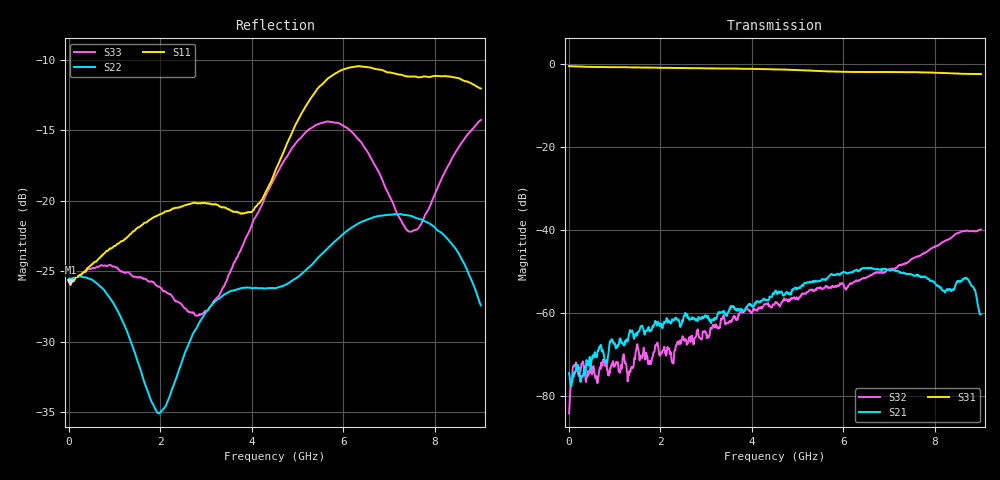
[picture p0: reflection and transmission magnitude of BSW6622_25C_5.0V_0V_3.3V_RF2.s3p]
!Agilent Technologies,N5230C,MY49001333,A.09.33.09
!Agilent N5230C: A.09.33.09
!Date: Monday, September 23, 2024 11:09:14
!Correction: S11(Full 3 Port(1,2,3))
!S12(Full 3 Port(1,2,3))
!S13(Full 3 Port(1,2,3))
!S21(Full 3 Port(1,2,3))
!S22(Full 3 Port(1,2,3))
!S23(Full 3 Port(1,2,3))
!S31(Full 3 Port(1,2,3))
!S32(Full 3 Port(1,2,3))
!S33(Full 3 Port(1,2,3))
!S3P File: Measurements: <S11,S12,S13>,
!<S21,S22,S23>,
!<S31,S32,S33>:
# Hz S  MA  R 50
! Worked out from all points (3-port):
!   901 points, 10 MHz to 9.01 GHz, reference 50 ohm
!   strongest paths, dB at 10 MHz, 2.26 GHz, 4.51 GHz, 6.76 GHz, 9.01 GHz:
!     S31: -0.6, -1.0, -1.3, -2.0, -2.5
!     S21: -74.4, -61.5, -54.7, -49.5, -60.2
!     S32: -84.1, -71.7, -57.6, -50.2, -39.9
!   lowest |S11| = -25.8 dB at 40 MHz (marker M1), VSWR 1.11, Z = 55.4 - j0.441 ohm
!   |S11| at or under -10 dB: start of sweep to end of sweep
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1e7  0.05148 -0.6  0.000127 11.6  0.9374 -2.5
     0.0001906 -47.2  0.05292 -1.2  9.816e-05 -60.5
     0.9373 -2.5  6.264e-05 -70.1  0.05153 -4.2
4e7  0.05144 -4.4  0.0001566 70.6  0.936 -4.7
     0.000147 -49.8  0.05296 -2.2  0.0001338 -132.6
     0.9357 -4.6  0.0001239 -5.2  0.05276 -3.4
1.6e9  0.08205 169.2  0.0006582 -76.7  0.9007 -167.9
       0.0007064 -62.9  0.02431 -139.4  0.0002741 -173.5
       0.9019 -168.0  0.0002947 -13.1  0.05339 175.8
2.63e9  0.0973 66.8  0.0008158 -164.1  0.8863 84.5
        0.0008561 -164.7  0.03112 48.7  0.0004149 -81.7
        0.8878 84.5  0.0004789 -99.8  0.04037 12.4
3.51e9  0.09318 -28.5  0.001184 124.7  0.8747 -7.6
        0.001109 116.3  0.04757 -35.9  0.0009936 -161.1
        0.8772 -7.5  0.0007874 -161.8  0.05504 -122.7
4.51e9  0.1269 174.8  0.001588 30.1  0.8544 -112.1
        0.00184 32.5  0.04891 -138.9  0.001185 91.4
        0.8583 -111.6  0.001322 86.1  0.1212 145.5
5.9e9  0.2879 16.2  0.002774 -114.9  0.817 103.8
       0.002971 -111.7  0.07364 69.3  0.002165 -43.7
       0.8043 104.2  0.002119 -43.9  0.1887 16.4
6.91e9  0.2881 -69.8  0.003599 133.6  0.8073 -1.5
        0.003385 133.9  0.08894 -21.5  0.003252 -132.4
        0.7975 -1.9  0.003096 -134.0  0.1128 -94.0
7.82e9  0.2761 -136.0  0.002444 46.8  0.7927 -98.1
        0.0027 46.3  0.0841 -102.0  0.00542 150.2
        0.7876 -98.2  0.005436 149.1  0.09076 111.0
9.01e9  0.2504 109.8  0.000926 -80.0  0.7601 135.7
        0.0009746 -87.0  0.04256 145.9  0.009808 19.9
        0.7538 134.5  0.01016 21.0  0.1937 -16.7
